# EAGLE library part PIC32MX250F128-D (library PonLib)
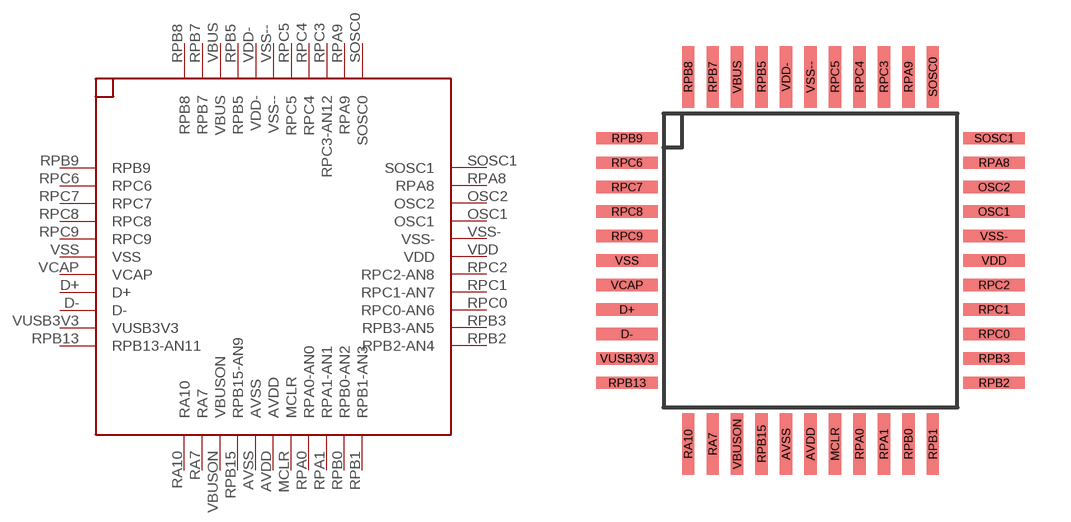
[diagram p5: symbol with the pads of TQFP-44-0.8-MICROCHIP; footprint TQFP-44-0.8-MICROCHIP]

Designator prefix -

## PIC32MX250F128-D  [TQFP-44-0.8-MICROCHIP]
AVDD  AVDD
AVSS  AVSS
D+  D+
D-  D-
MCLR  MCLR
OSC1  OSC1
OSC2  OSC2
RA7  RA7
RA10  RA10
RPA0  RPA0-AN0
RPA1  RPA1-AN1
RPA8  RPA8
RPA9  RPA9
RPB0  RPB0-AN2
RPB1  RPB1-AN3
RPB2  RPB2-AN4
RPB3  RPB3-AN5
RPB5  RPB5
RPB7  RPB7
RPB8  RPB8
RPB9  RPB9
RPB13  RPB13-AN11
RPB15  RPB15-AN9
RPC0  RPC0-AN6
RPC1  RPC1-AN7
RPC2  RPC2-AN8
RPC3  RPC3-AN12
RPC4  RPC4
RPC5  RPC5
RPC6  RPC6
RPC7  RPC7
RPC8  RPC8
RPC9  RPC9
SOSC0  SOSC0
SOSC1  SOSC1
VBUS  VBUS
VBUSON  VBUSON
VCAP  VCAP
VDD  VDD
VDD-  VDD-
VSS  VSS
VSS-  VSS-
VSS--  VSS--
VUSB3V3  VUSB3V3

## Footprint TQFP-44-0.8-MICROCHIP (pad centres in mm)
smd 0.4 x 2: AVDD 0,-6; AVSS -0.8,-6; MCLR 0.8,-6; RA7 -3.2,-6; RA10 -4,-6; RPA0 1.6,-6; RPA1 2.4,-6; RPA9 3.2,6; RPB0 3.2,-6; RPB1 4,-6; RPB5 -1.6,6; RPB7 -3.2,6; RPB8 -4,6; RPB15 -1.6,-6; RPC3 2.4,6; RPC4 1.6,6; RPC5 0.8,6; SOSC0 4,6; VBUS -2.4,6; VBUSON -2.4,-6; VDD- -0.8,6; VSS-- 0,6
smd 2 x 0.4: D+ -6,-1.6; D- -6,-2.4; OSC1 6,1.6; OSC2 6,2.4; RPA8 6,3.2; RPB2 6,-4; RPB3 6,-3.2; RPB9 -6,4; RPB13 -6,-4; RPC0 6,-2.4; RPC1 6,-1.6; RPC2 6,-0.8; RPC6 -6,3.2; RPC7 -6,2.4; RPC8 -6,1.6; RPC9 -6,0.8; SOSC1 6,4; VCAP -6,-0.8; VDD 6,0; VSS -6,0; VSS- 6,0.8; VUSB3V3 -6,-3.2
